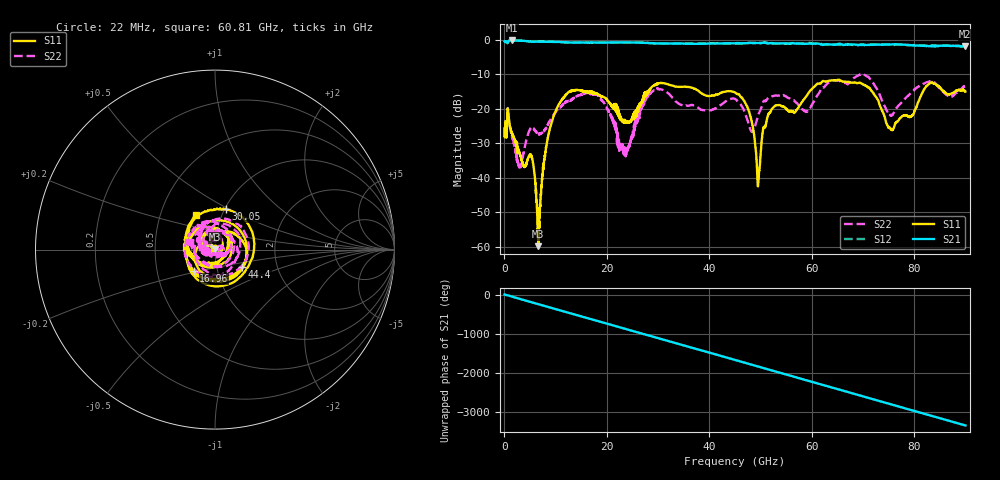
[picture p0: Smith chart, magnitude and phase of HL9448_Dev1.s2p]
! 5/9/2022 12:32:21 PM
! C:\USERS\VECTORSTARUSER\DESKTOP\JASON\HL9449-11\HL9449-11-NE01.S2P
! CHANNEL.1
! TR.MEASUREMENT
! CORRECTED.DATA
# GHZ S RI R 50.0
! FREQ.GHZ  S11RE  S11IM  S21RE  S21IM  S12RE  S12IM  S22RE  S22IM
!; PortSelection: Port_12
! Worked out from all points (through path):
!   4091 points, 22 MHz to 90 GHz, reference 50 ohm
!   highest |S21| = -0.26 dB at 1.386 GHz (marker M1); lowest = -2.0 dB at 89.96 GHz (marker M2)
!   group delay of S21, straight-line fit = 103 ps
!   lowest |S11| = -59.8 dB at 6.6 GHz (marker M3), VSWR 1.00, Z = 50 + j0.102 ohm
!   |S11| at or under -10 dB: start of sweep to end of sweep
!   |S22| runs from -37.4 to -9.8 dB; largest |S21 - S12| = 0.046
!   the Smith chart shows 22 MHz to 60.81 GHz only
!   S11 on the Smith chart (normalised r, x): 22 MHz: 0.90, -0.01; 16.96 GHz: 0.77, -0.19; 30.05 GHz: 1.01, +0.48; 44.4 GHz: 1.33, -0.26; 60.81 GHz: 0.76, +0.31
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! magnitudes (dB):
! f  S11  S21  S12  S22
! 22 MHz  -25.6  -0.5  -0.5  -25.5
! 1.386 GHz  -27.0  -0.3  -0.3  -27.8
! 3.036 GHz  -33.5  -0.3  -0.3  -37.4
! 5.302 GHz  -33.9  -0.6  -0.6  -25.4
! 6.6 GHz  -59.8  -0.6  -0.6  -27.4
! 9.57 GHz  -22.2  -0.7  -0.7  -21.8
! 15.03 GHz  -14.8  -0.9  -0.9  -16.0
! 16.96 GHz  -15.5  -0.9  -0.9  -15.9
! 23.65 GHz  -23.6  -0.8  -0.8  -33.3
! 30.03 GHz  -12.7  -1.1  -1.1  -14.4
! 30.05 GHz  -12.7  -1.1  -1.1  -14.4
! 44.4 GHz  -15.0  -1.1  -1.1  -17.1
! 45.01 GHz  -15.3  -1.1  -1.1  -17.1
! 47.83 GHz  -21.1  -1.0  -0.9  -25.2
! 49.59 GHz  -40.9  -1.0  -1.0  -21.6
! 51.92 GHz  -21.0  -1.0  -1.2  -16.7
! 60.02 GHz  -14.3  -1.2  -1.1  -18.9
! 60.81 GHz  -13.1  -1.2  -1.2  -16.8
! 70 GHz  -13.0  -1.5  -1.4  -9.9
! 75.02 GHz  -25.6  -1.4  -1.5  -21.5
! 89.96 GHz  -15.0  -2.0  -1.8  -13.4
! 90 GHz  -15.0  -2.0  -1.8  -13.4
